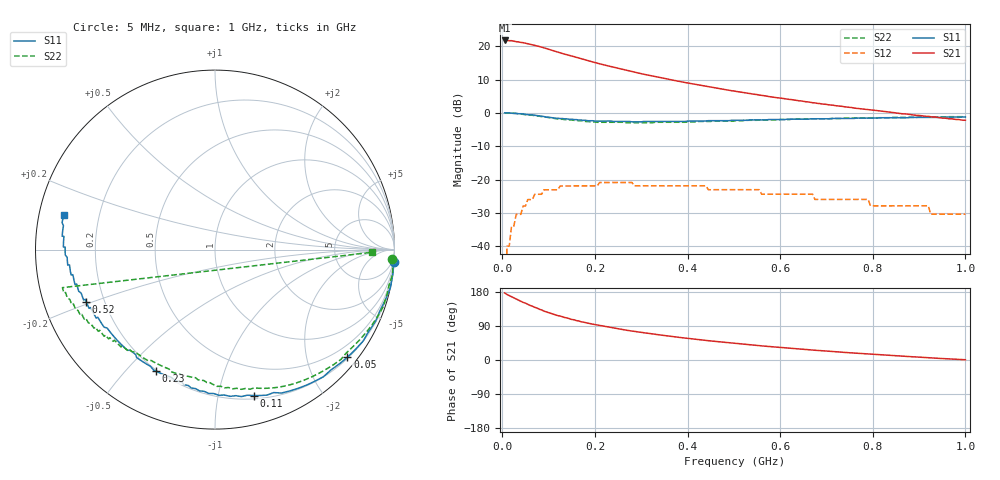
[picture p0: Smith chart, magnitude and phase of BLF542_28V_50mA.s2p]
! Filename:  BLF542_28V_50mA.s2p
! Philips part #: BLF542  ! Created Thu Apr  3 15:35:15 2003
# hz S ma R 50
! 2 Port Network Data from SP1.SP block
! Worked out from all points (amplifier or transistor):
!   200 points, 5 MHz to 1 GHz, reference 50 ohm
!   highest |S21| = 21.7 dB at 5 MHz (marker M1)
!   |S21| within 3 dB of that: start of sweep to 108 MHz
!   S11 on the Smith chart (normalised r, x): 5 MHz: -0, -28; 50 MHz: 0.22, -2.80; 110 MHz: 0.23, -1.27; 230 MHz: 0.19, -0.61; 520 MHz: 0.13, -0.19; 1 GHz: 0.07, +0.11
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5000000  1 -4.1  12.2 177.0  0 0.0  0.99 -3.2
1e7  1 -8.2  12.2 173.0  0.01 83.5  1 -7.8
1.5e7  1 -12.1  12.1 170.0  0.01 80.7  0.99 -11.3
2e7  0.99 -16.3  12.1 167.0  0.02 78.1  0.99 -14.5
3.5e7  0.97 -28.0  11.6 158.0  0.03 68.8  0.97 -25.7
4.5e7  0.96 -35.4  11.3 152.0  0.04 63.5  0.95 -32.0
5e7  0.951 -39.1  11.1 150.0  0.04 60.9  0.94 -35.1
6e7  0.931 -46.1  10.7 144.0  0.05 55.8  0.931 -41.1
8e7  0.901 -59.1  9.92 134.0  0.0601 46.2  0.891 -52.7
9e7  0.881 -65.1  9.47 129.0  0.0701 41.6  0.871 -58.4
1.1e8  0.841 -75.2  8.55 121.0  0.0701 33.5  0.831 -68.2
1.5e8  0.802 -92.5  7.12 107.0  0.0802 21.2  0.782 -82.8
1.75e8  0.772 -101.0  6.37 99.9  0.0802 14.2  0.752 -90.7
2.3e8  0.753 -116.0  5.04 86.9  0.0903 2.7  0.722 -104.0
2.7e8  0.743 -125.0  4.33 78.2  0.0903 -4.9  0.713 -111.0
3.4e8  0.743 -137.0  3.4 66.2  0.0803 -14.8  0.723 -122.0
5.05e8  0.774 -156.0  2.1 43.6  0.0703 -32.7  0.764 -138.0
5.2e8  0.774 -158.0  2.02 41.9  0.0703 -33.9  0.764 -140.0
6.7e8  0.814 -171.0  1.42 26.2  0.0603 -44.6  0.815 -150.0
8.35e8  0.845 178.0  1.03 12.3  0.0402 -51.6  0.845 -159.0
9.95e8  0.866 168.0  0.775 1.1  0.0302 -52.9  0.876 -166.0
1e9  0.866 167.0  0.775 0.7  0.0302 -52.8  0.876 -1.0
